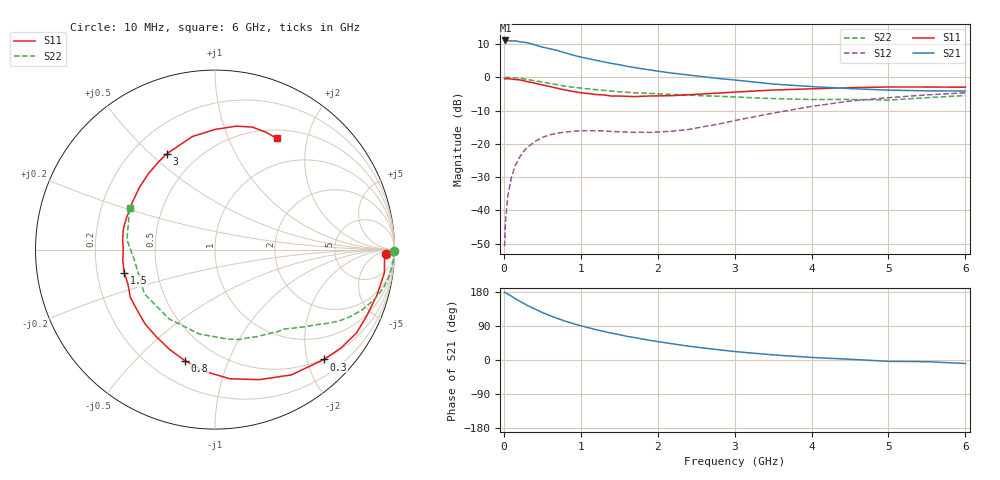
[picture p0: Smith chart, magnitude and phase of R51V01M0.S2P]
! SIEMENS Small Signal Semiconductors
! BFR183
! Si NPN RF Bipolar Junction Transistor in SOT23
! VCE = 1 V  IC = 1 mA
! Common Emitter S-Parameters:  May  1996
# GHz  S  MA  R  50
!  f  S11  S21  S12  S22
! GHz  MAG  ANG  MAG  ANG  MAG  ANG  MAG  ANG
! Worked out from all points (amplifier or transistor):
!   36 points, 10 MHz to 6 GHz, reference 50 ohm
!   highest |S21| = 11.0 dB at 20 MHz (marker M1)
!   |S21| within 3 dB of that: start of sweep to 692.6 MHz
!   unconditionally stable (mu >= 1): 1.609 GHz to 3.204 GHz
!   at 250 MHz: K = 0.16, MSG = 16.5 dB, |S12| = -22.5 dB
!   at 1.4 GHz: K = 0.87, MSG = 10.2 dB, |S12| = -16.3 dB
!   at 6 GHz: K = 0.98, MSG = 0.3 dB, |S12| = -4.7 dB
!   S11 on the Smith chart (normalised r, x): 10 MHz: 31, -17; 300 MHz: 0.48, -2.32; 800 MHz: 0.34, -0.71; 1.5 GHz: 0.32, -0.11; 3 GHz: 0.34, +0.57; 6 GHz: 0.61, +1.52
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0.01  0.9518 -1.6  3.493 179.2  0.0029 90.9  0.9984 -0.6
0.02  0.946 -3.2  3.568 177.5  0.0065 88.5  0.992 -1.3
0.05  0.9528 -7.8  3.554 174.1  0.0159 84.9  0.996 -3.2
0.1  0.9374 -15.6  3.508 168.4  0.032 80.5  0.988 -6.2
0.15  0.923 -23.2  3.518 161.5  0.0474 75.8  0.9783 -9.4
0.3  0.8625 -45.2  3.307 144.5  0.0874 63.6  0.9283 -17.6
0.4  0.8177 -58.6  3.079 135.0  0.1076 55.9  0.8854 -22.3
0.5  0.7657 -71.1  2.83 125.3  0.1247 49.8  0.846 -25.9
0.6  0.7246 -83.4  2.68 117.0  0.1366 44.2  0.8061 -29.2
0.7  0.6813 -94.7  2.514 109.4  0.1447 39.7  0.7688 -31.9
0.8  0.6415 -105.1  2.324 102.4  0.1502 35.9  0.7343 -34.3
0.9  0.6116 -114.3  2.149 96.1  0.1546 32.9  0.7073 -36.2
1.1  0.5688 -133.2  1.901 85.2  0.1574 28.4  0.6672 -39.9
1.3  0.5415 -150.6  1.701 75.3  0.1563 25.9  0.634 -43.1
1.5  0.5217 -165.7  1.545 66.8  0.1509 25.9  0.6048 -46.4
1.9  0.5227 167.7  1.287 52.0  0.1483 31.0  0.5726 -53.4
2.2  0.5299 151.0  1.148 42.5  0.1551 37.8  0.5498 -59.2
3  0.5981 116.5  0.909 22.3  0.2231 49.5  0.5048 -81.5
3.5  0.6424 101.3  0.791 13.5  0.289 48.1  0.4785 -100.5
4.5  0.6977 80.3  0.675 1.9  0.4389 35.0  0.4641 -148.0
5.5  0.7127 66.3  0.624 -4.5  0.5433 18.7  0.4933 173.7
6  0.7088 60.9  0.621 -9.2  0.5827 9.1  0.5302 153.8
